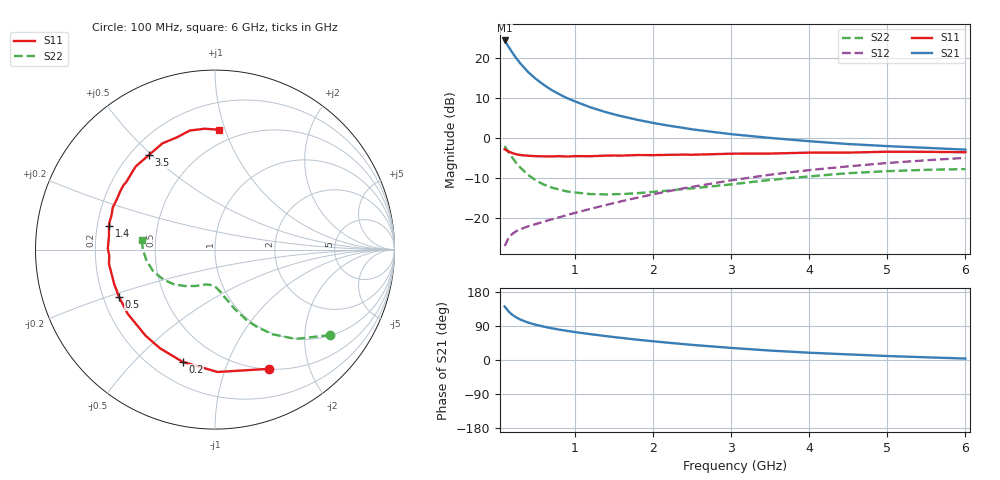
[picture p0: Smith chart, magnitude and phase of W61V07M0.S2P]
! SIEMENS Small Signal Semiconductors
! BFR193W
! Si NPN RF Bipolar Junction Transistor in SOT323
! VCE = 1 V  IC = 7 mA
! Common Emitter S-Parameters:  September  1992
# GHz  S  MA  R  50
!  f  S11  S21  S12  S22
! GHz  MAG  ANG  MAG  ANG  MAG  ANG  MAG  ANG
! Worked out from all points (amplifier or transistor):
!   28 points, 100 MHz to 6 GHz, reference 50 ohm
!   highest |S21| = 24.5 dB at 100 MHz (marker M1)
!   |S21| within 3 dB of that: start of sweep to 197.6 MHz
!   unconditionally stable (mu >= 1): 1.058 GHz to 2.752 GHz
!   at 300 MHz: K = 0.46, MSG = 20.8 dB, |S12| = -22.8 dB
!   at 1.5 GHz: K = 1.07, MAG = 9.5 dB, |S12| = -16.2 dB
!   at 6 GHz: K = 0.95, MSG = 1.0 dB, |S12| = -4.9 dB
!   S11 on the Smith chart (normalised r, x): 100 MHz: 0.50, -1.42; 200 MHz: 0.32, -0.70; 500 MHz: 0.27, -0.22; 1.4 GHz: 0.25, +0.10; 3.5 GHz: 0.27, +0.49; 6 GHz: 0.39, +0.95
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0.1  0.7286 -65.8  16.77 141.3  0.0445 59.5  0.799 -36.6
0.15  0.682 -88.8  13.99 128.4  0.0563 51.4  0.6706 -47.9
0.2  0.651 -106.0  11.77 119.0  0.0635 46.3  0.5694 -55.9
0.25  0.6296 -119.0  10.02 112.3  0.0687 43.6  0.4877 -61.7
0.3  0.6164 -128.8  8.681 106.9  0.0725 42.3  0.4307 -65.8
0.4  0.6037 -143.7  6.767 98.8  0.0788 41.8  0.3479 -71.7
0.5  0.5962 -153.5  5.533 92.9  0.0842 42.8  0.2967 -75.7
0.6  0.5935 -161.1  4.672 88.1  0.0902 44.4  0.2635 -79.4
0.7  0.5919 -167.1  4.027 83.8  0.0963 46.1  0.2418 -82.0
0.8  0.5961 -172.3  3.56 80.1  0.1023 47.9  0.2271 -84.8
0.9  0.5898 -176.6  3.181 76.8  0.1092 49.6  0.2157 -86.9
1  0.5971 179.4  2.894 73.7  0.1161 51.1  0.2093 -89.2
1.2  0.5956 172.8  2.438 68.2  0.1305 53.5  0.1998 -94.3
1.4  0.6057 167.3  2.117 63.0  0.1461 55.3  0.1982 -98.7
1.8  0.6159 157.6  1.702 53.6  0.1801 57.7  0.2051 -107.5
2.2  0.6196 148.7  1.438 45.5  0.2172 58.2  0.221 -114.9
2.5  0.6214 142.9  1.293 39.9  0.2464 57.6  0.2356 -120.5
3  0.6402 133.6  1.125 31.9  0.2969 55.5  0.2644 -129.9
3.5  0.6428 125.0  1.009 24.9  0.3494 52.2  0.3004 -140.1
4.5  0.6607 108.5  0.846 14.8  0.4445 43.8  0.365 -160.7
5.5  0.6758 94.8  0.758 7.1  0.5304 34.3  0.4023 179.8
6  0.6684 88.2  0.72 3.8  0.5678 29.1  0.4107 172.9
